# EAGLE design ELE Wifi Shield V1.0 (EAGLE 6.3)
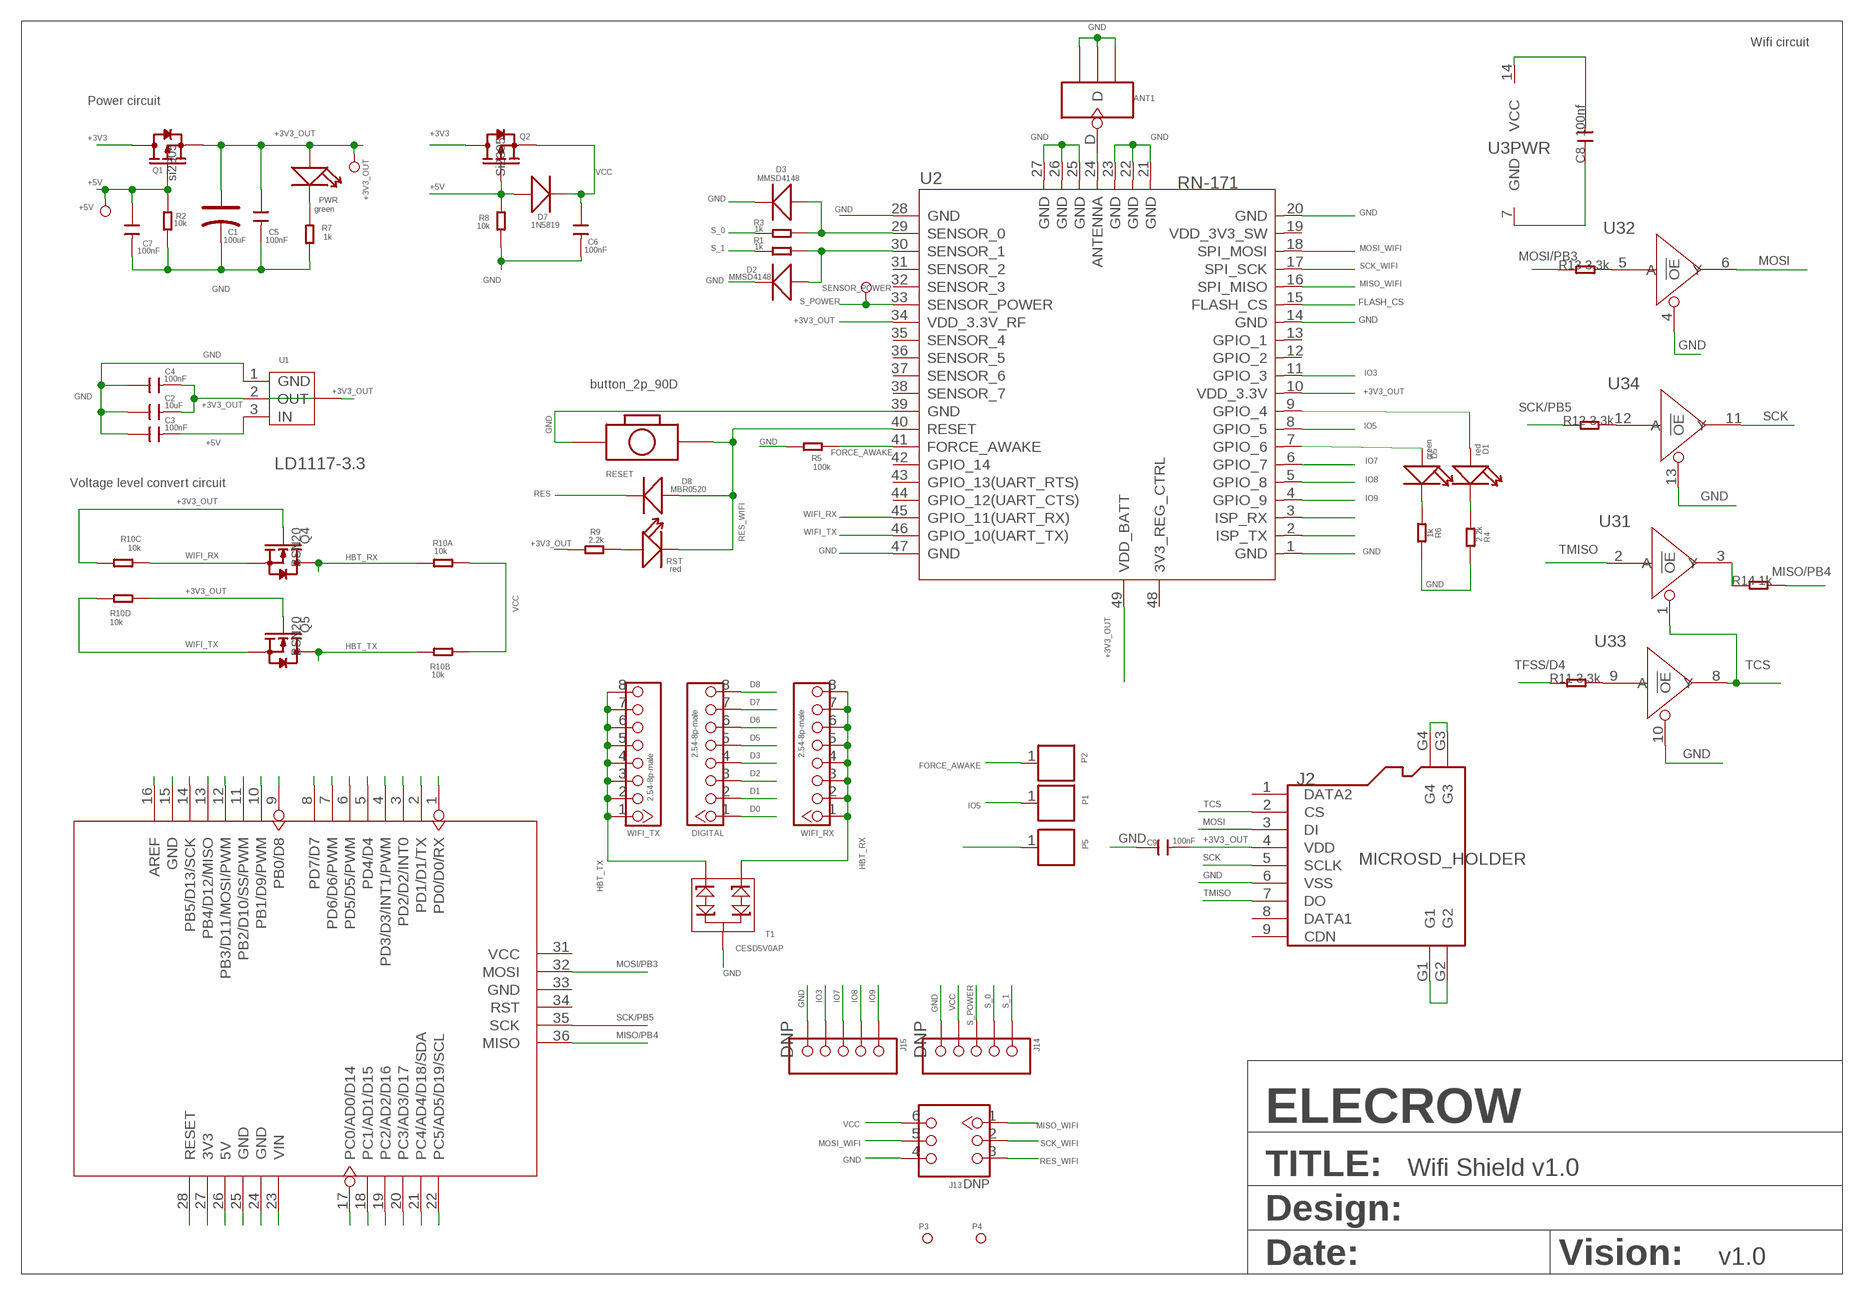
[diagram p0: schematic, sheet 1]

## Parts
+3V3_OUT  PAD-TEST-POINT-CIRCLE_SIZE_3030  [TP_3535]
+5V  PAD-TEST-POINT-CIRCLE_SIZE_3030  [TP_3535]
ANT1  ANTENNA-U-FL  [4P-U-FL]
C1  100uF  CAP-AVX-B  [AVX-B]
C2  10uF  C-0603  [C0603]
C3  100nF  C-0603  [C0603]
C4  100nF  C-0603  [C0603]
C5  100nF  C-0603  [C0603]
C6  100nF  C-0603  [C0603]
C7  100nF  C-0603  [C0603]
C8  100nf  C-0603  [C0603]
C9  100nF  C-0603  [C0603]
D1  red  LED'0603'  [LED-0603]
D2  MMSD4148  D-MBR0520LT1  [SOD123-2.7X1.6]
D3  MMSD4148  D-MBR0520LT1  [SOD123-2.7X1.6]
D5  green  LED'0603'  [LED-0603]
D7  1N5819  D-SMA  [D2010]
D8  MBR0520  D-MBR0520LT1  [SOD123-2.7X1.6]
DIGITAL  2.54-8p-male  HEADER-8P-2.54  [8P-2.54]
J2  MICROSD_HOLDER  HOLDER-MICROSD-9P  [9P-SMD-W/-RING]
J13  DNP  HEADER-2X3P-2.54  [2X3P-2.54]
J14  DNP  HEADER-5P-2.54  [5P-2.54]
J15  DNP  HEADER-5P-2.54  [5P-2.54]
P1  DNP  PAD'60/30'  [1P-65/35MIL]
P2  DNP  PAD'60/30'  [1P-65/35MIL]
P3  PAD-MARK  [ROUND-MARK-1.0]
P4  PAD-MARK  [ROUND-MARK-1.0]
P5  DNP  PAD'60/30'  [1P-65/35MIL]
PWR  green  LED'0603'  [LED-0603]
Q1  si2305  MOSFET-P'SI2323CDS/SI2305DS<BR>'  [SOT23]
Q2  Si2305  MOSFET-P'SI2323CDS/SI2305DS<BR>'  [SOT23]
Q4  BSN20  MOSFET-N'SOT23'  [SOT23]
Q5  BSN20  MOSFET-N'SOT23'  [SOT23]
R1  1k  R-0603  [R0603]
R2  10k  R-0603  [R0603]
R3  1k  R-0603  [R0603]
R4  2.2k  R-0603  [R0603]
R5  100k  R-0603  [R0603]
R6  1k  R-0603  [R0603]
R7  1k  R-0603  [R0603]
R8  10k  R-0603  [R0603]
R9  2.2k  R-0603  [R0603]
R10  10k  005-4R_1206  [R1206-8]
R11  3.3k  R-0603  [R0603]
R12  3.3k  R-0603  [R0603]
R13  3.3k  R-0603  [R0603]
R14  1k  R-0603  [R0603]
RESET  button_2p_90D  BOTTON-2P-90  [2P-7.62X3.56-90D]
RST  red  LED'0603'  [LED-0603]
SENSOR_POWER  PAD-TEST-POINT-CIRCLE_SIZE_3030  [TP_3535]
T1  CESD5V0AP  D-ESD-PESDXL2BT  [SOT23]
U1  LD1117-3.3  LD1117SOT89  [SOT89]
U2  RN-171  WIFI-RN-171  [49P-1.27-26.67X17.78]
U3  74VHC125PW  [TSSOP14]
U4  long female pin_8*2_6*2_2X3  ARDUINO  [ARDUINO]
WIFI_RX  2.54-8p-male  HEADER-8P-2.54  [8P-2.54]
WIFI_TX  2.54-8p-male  HEADER-8P-2.54  [8P-2.54]

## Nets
+3V3: Q1.3(D) Q2.3(D) U4.27(3V3)
+3V3_OUT: +3V3_OUT.T C1.+ C2.2 C4.2 C5.1 C9.2 J2.4(VDD) PWR.+ Q1.2(S) Q4.1(G) Q5.1(G) R9.2 R10.5 R10.6 U1.2(OUT) U1.4(TAB) U2.10(VDD_3.3V) U2.34(VDD_3.3V_RF) U2.49(VDD_BATT)
+5V: +5V.T C3.2 C7.1 D7.+ Q1.1(G) Q2.1(G) R2.1 R8.1 U1.3(IN) U4.26(5V)
A0: U4.17(PC0/AD0/D14)
A1: U4.18(PC1/AD1/D15)
A2: U4.19(PC2/AD2/D16)
A3: U4.20(PC3/AD3/D17)
A4: U4.21(PC4/AD4/D18/SDA)
A5: U4.22(PC5/AD5/D19/SCL)
AREF: U4.16(AREF)
D0: DIGITAL.1 U4.1(PD0/D0/RX)
D1: DIGITAL.2 U4.2(PD1/D1/TX)
D2: DIGITAL.3 U4.3(PD2/D2/INT0)
D3: DIGITAL.4 U4.4(PD3/D3/INT1/PWM)
D5: DIGITAL.5 U4.6(PD5/D5/PWM)
D6: DIGITAL.6 U4.7(PD6/D6/PWM)
D7: DIGITAL.7 U4.8(PD7/D7)
D8: DIGITAL.8 U4.9(PB0/D8)
D9: U4.10(PB1/D9/PWM)
D10: U4.11(PB2/D10/SS/PWM)
D11: U4.12(PB3/D11/MOSI/PWM)
D12: U4.13(PB4/D12/MISO)
D13: U4.14(PB5/D13/SCK)
FLASH_CS: P5.1 U2.15(FLASH_CS)
FORCE_AWAKE: P2.1 R5.1 U2.41(FORCE_AWAKE)
GND: ANT1.GND1 ANT1.GND2 ANT1.GND3 C1.- C2.1 C3.1 C4.1 C5.2 C6.2 C7.2 C8.1 C9.1 D2.1(-) D3.1(-) J2.6(VSS) J2.G1 J2.G2 J2.G3 J2.G4 J13.4 J14.5 J15.5 R2.2 R4.1 R5.2 R6.1 R7.1 R8.2 RESET.P$2 T1.3 U1.1(GND) U2.1(GND) U2.14(GND) U2.20(GND) U2.21(GND) U2.22(GND) U2.23(GND) U2.25(GND) U2.26(GND) U2.27(GND) U2.28(GND) U2.39(GND) U2.47(GND) U3.4(2:!OE) U3.7(PWR:GND) U3.10(3:!OE) U3.13(4:!OE) U4.15(GND) U4.24(GND) U4.25(GND)
HBT_RX: Q4.3(D) R10.1 T1.1 WIFI_RX.1 WIFI_RX.2 WIFI_RX.3 WIFI_RX.4 WIFI_RX.5 WIFI_RX.6 WIFI_RX.7 WIFI_RX.8
HBT_TX: Q5.3(D) R10.2 T1.2 WIFI_TX.1 WIFI_TX.2 WIFI_TX.3 WIFI_TX.4 WIFI_TX.5 WIFI_TX.6 WIFI_TX.7 WIFI_TX.8
IO3: J15.4 U2.11(GPIO_3)
IO5: P1.1 U2.8(GPIO_5)
IO7: J15.3 U2.6(GPIO_7)
IO8: J15.2 U2.5(GPIO_8)
IO9: J15.1 U2.4(GPIO_9)
MISO/PB4: R14.2 U4.36(MISO)
MISO_WIFI: J13.1 U2.16(SPI_MISO)
MOSI: J2.3(DI) U3.6(2:Y)
MOSI/PB3: R13.1 U4.32(MOSI)
MOSI_WIFI: J13.5 U2.18(SPI_MOSI)
N$1: R9.1 RST.+
N$2: D3.2(+) R3.1 U2.29(SENSOR_0)
N$3: D2.2(+) R1.1 U2.30(SENSOR_1)
N$6: R13.2 U3.5(2:A)
N$8: R12.2 U3.12(4:A)
N$10: U2.2(ISP_TX)
N$11: U2.3(ISP_RX)
N$12: R11.2 U3.9(3:A)
N$15: D5.+ U2.7(GPIO_6)
N$16: R14.1 U3.3(1:Y)
N$20: ANT1.D U2.24(ANTENNA)
N$22: D1.+ U2.9(GPIO_4)
N$23: D5.- R6.2
N$25: D1.- R4.2
N$26: PWR.- R7.2
RES: D8.1(-) U4.28(RESET)
RES_WIFI: D8.2(+) J13.3 RESET.P$1 RST.- U2.40(RESET)
S_0: J14.2 R3.2
S_1: J14.1 R1.2
S_POWER: J14.3 SENSOR_POWER.T U2.33(SENSOR_POWER)
SCK: J2.5(SCLK) U3.11(4:Y)
SCK/PB5: R12.1 U4.35(SCK)
SCK_WIFI: J13.2 U2.17(SPI_SCK)
TCS: J2.2(CS) U3.1(1:!OE) U3.8(3:Y)
TFSS/D4: R11.1 U4.5(PD4/D4)
TMISO: J2.7(DO) U3.2(1:A)
VCC: C6.1 C8.2 D7.- J13.6 J14.4 Q2.2(S) R10.7 R10.8 U3.14(PWR:VCC)
VIN: U4.23(VIN)
WIFI_RX: Q4.2(S) R10.3 U2.45(GPIO_11(UART_RX))
WIFI_TX: Q5.2(S) R10.4 U2.46(GPIO_10(UART_TX))
Unconnected: J2.1(DATA2) J2.8(DATA1) J2.9(CDN) U2.12(GPIO_2) U2.13(GPIO_1) U2.19(VDD_3V3_SW) U2.31(SENSOR_2) U2.32(SENSOR_3) U2.35(SENSOR_4) U2.36(SENSOR_5) U2.37(SENSOR_6) U2.38(SENSOR_7) U2.42(GPIO_14) U2.43(GPIO_13(UART_RTS)) U2.44(GPIO_12(UART_CTS)) U2.48(3V3_REG_CTRL) U4.31(VCC) U4.33(GND) U4.34(RST)

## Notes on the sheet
- Wifi circuit
- Power circuit
- Voltage level convert circuit
- ELECROW
- TITLE: | Wifi Shield v1.0
- Design:
- Date: | Vision: | v1.0

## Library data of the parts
+3V3_OUT +5V SENSOR_POWER = Discrete:PAD-TEST-POINT-CIRCLE
ANT1 = Connector:ANTENNA-U-FL
C1 = Discrete:CAP*: Electrolytic Capacitors,Tantalum Capacitors and Super Capacitors
C2-C9 = Discrete:C*: Ceramic Capacitors
D1 D5 PWR RST = Discrete:LED*
D2 D3 D7 D8 = Discrete:D*
DIGITAL WIFI_RX WIFI_TX = Connector:HEADER-8P
J2 = Connector:HOLDER-MICROSD-9P
J13 = Connector:HEADER-2X3P
J14 J15 = Connector:HEADER-5P
P1 P2 P5 = Discrete:PAD
P3 P4 = Discrete:PAD-MARK; PARTNO: DNP
Q1 Q2 = Discrete:MOSFET-P
Q4 Q5 = Discrete:MOSFET-N: IRLL014: http://www.vishay.com/docs/91319/sihll014.pdf
R1-R9 R11-R14 = Discrete:R*
R10 = Discrete:005-4R*: Resistor Array
RESET = Discrete:BOTTON-2P
T1 = Discrete:D-ESD-PESDXL2BT
U1 = IC:LD1117: Low Drop Fixed And Adjustable Positive Voltage Regulators http://www.datasheetcatalog.org/datasheet/SGSThomsonMicroelectronics/mXuqtqv.pdf
U2 = Module:WIFI-RN-171: WIFLY GSX 802.11 b/g wireless LAN Module
U3 = template:74V*125: Quad Buffer/Line Driver;3-state
U4 = moudle:ARDUINO

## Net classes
0 default: width 0.003 mm, drill 0.254 mm, clearance 0.152 mm

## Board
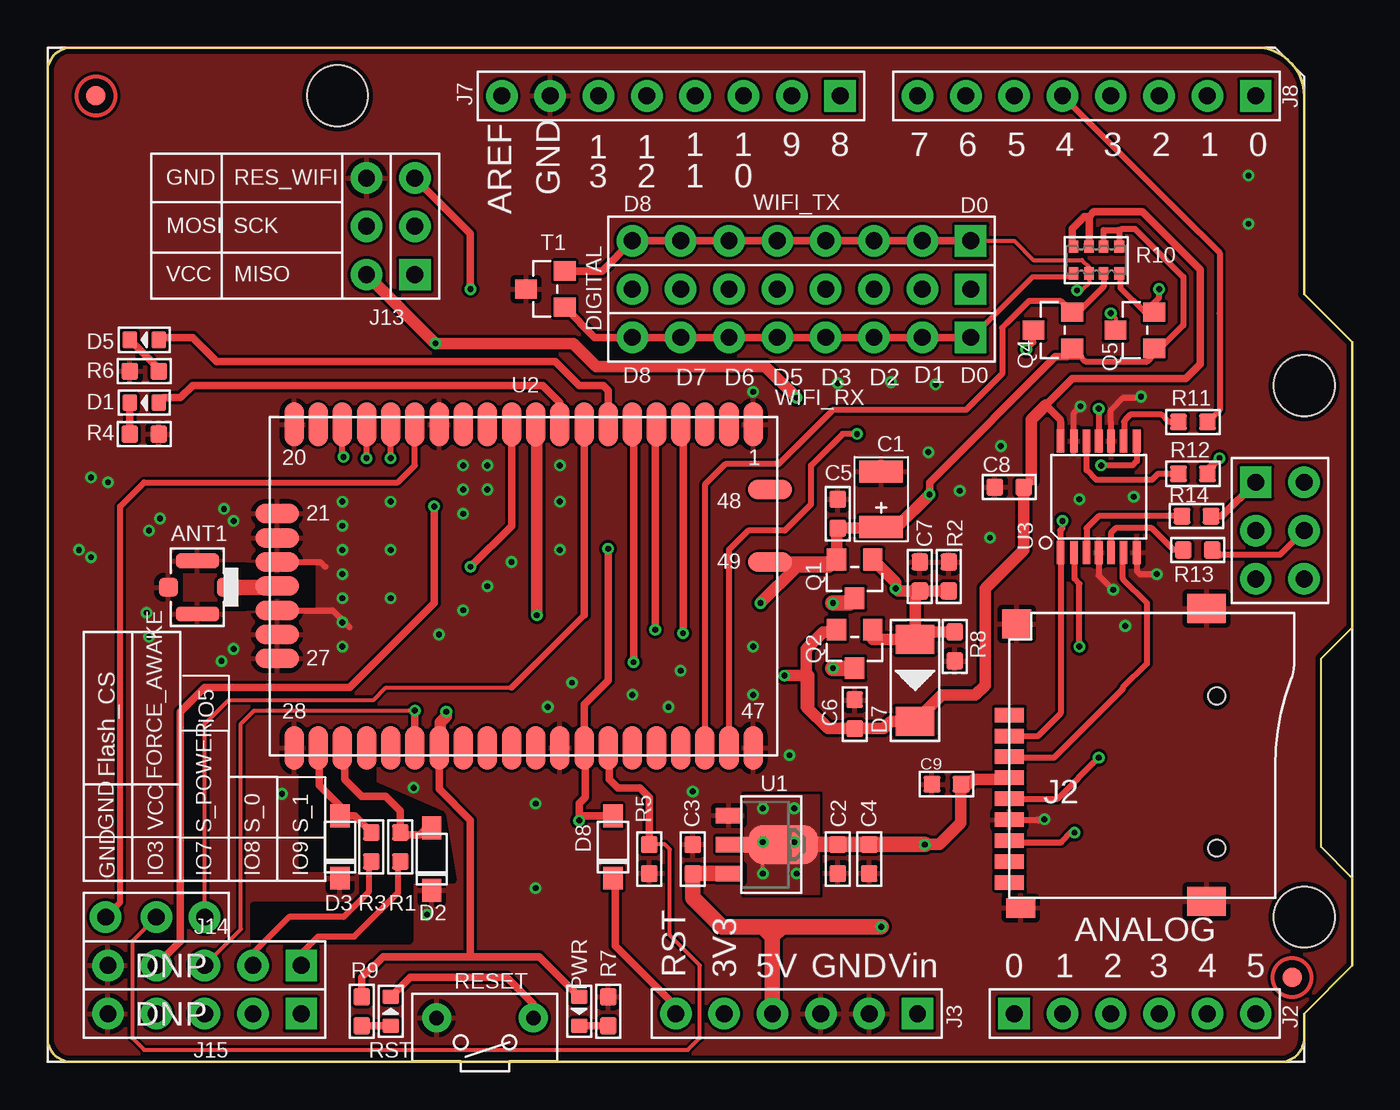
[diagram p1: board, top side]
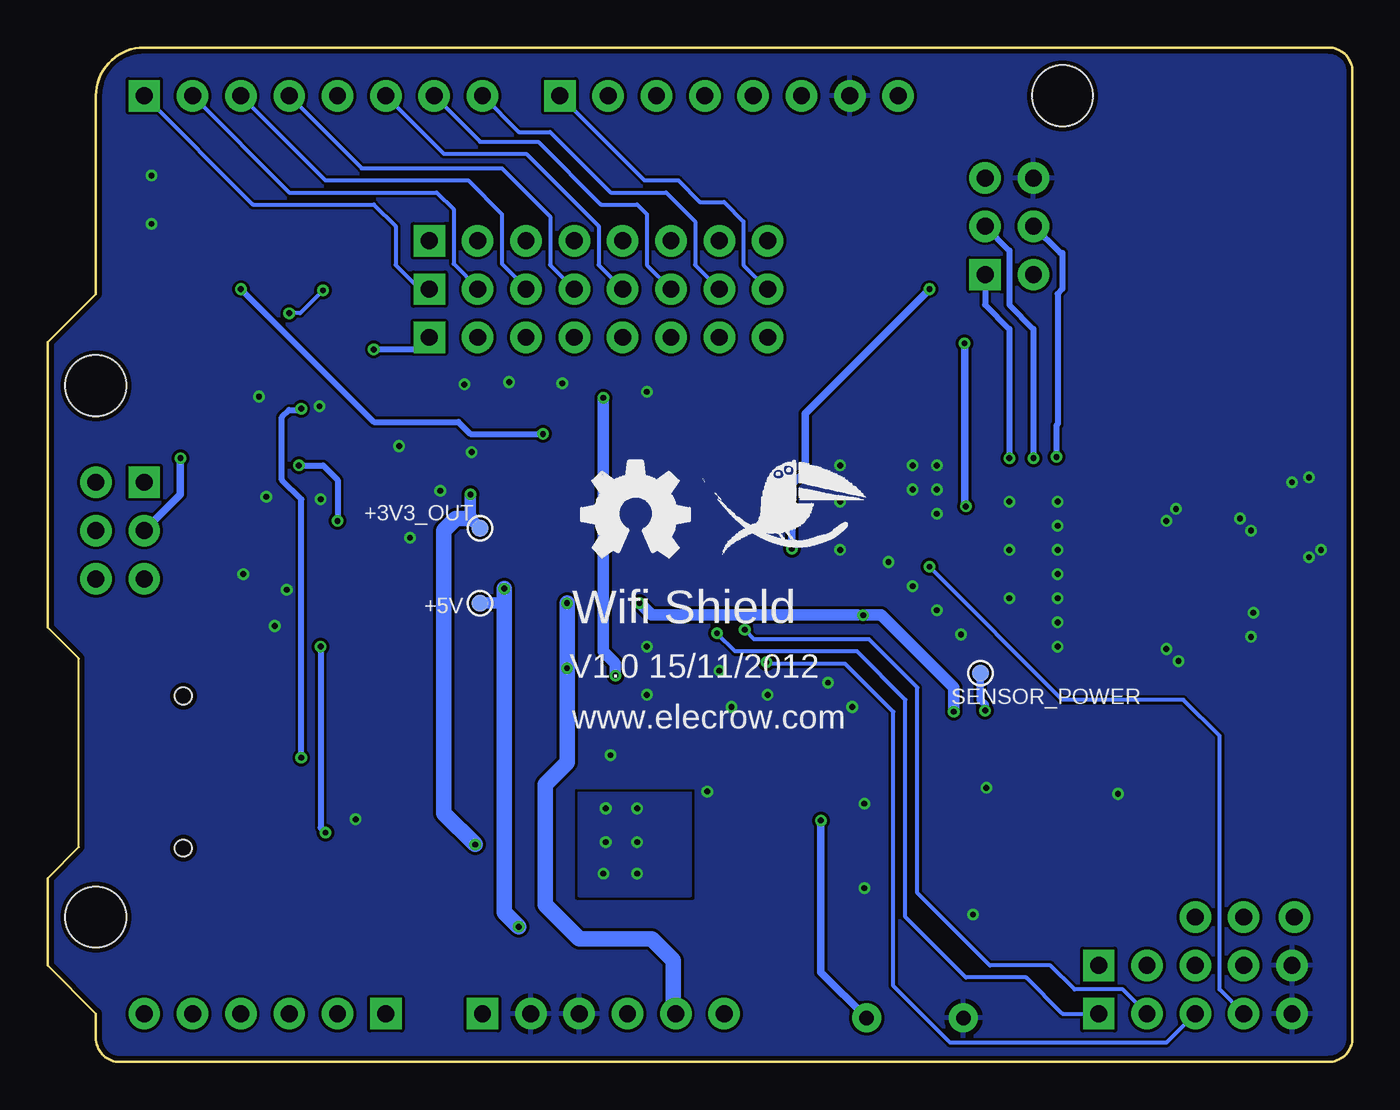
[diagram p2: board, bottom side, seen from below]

Size 68.58 x 53.34 mm. Coordinates in mm from the lower left corner, seen from the top.
Outline: 1.27,53.34 63.5,53.34 arc-90 66.04,50.8 66.04,40.39 68.58,37.85 68.58,22.86 66.93,21.21 66.93,11.3 68.58,9.65 68.58,5.08 66.04,2.54 66.04,1.27 arc-90 64.77,0 1.27,0 arc-90 0,1.27 0,52.07 arc-90 1.27,53.34
Copper layers (1*16): Top 0.035mm / dielectric 1.5mm / Bottom 0.035mm
Design rules "default": minimum track width 6mil, minimum drill 12mil, track to track 6mil, track to pad 6mil, pad to pad 6mil, via to via 6mil, smd to smd 0mil, copper to edge 10mil, drill to drill 10mil, minimum pad ring 10mil, minimum via ring 6mil, stop-mask expansion 2mil, vias tented up to drill 32mil, thermal gap 10mil
tRestrict: 16 lines

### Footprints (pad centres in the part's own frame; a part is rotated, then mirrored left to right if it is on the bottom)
TP_3535 = smd 0.889 x 0.889: T 0,0
4P-U-FL = smd 1.016 x 1.016: D -1.524,0; GND3 1.524,0 | smd 2.286 x 0.762: GND1 0,1.397; GND2 0,-1.397
AVX-B = smd 1.143 x 2.286: + -1.46,0; - 1.46,0
C0603 = smd 0.889 x 0.889: 1 -0.762,0; 2 0.762,0
LED-0603 = smd 0.762 x 0.889: + -0.762,0; - 0.762,0
SOD123-2.7X1.6 = smd 1.2 x 1.02: 1 -1.635,0; 2 1.635,0
D2010 = smd 1.524 x 2.032: + -2.159,0; - 2.159,0
8P-2.54 = drill 0.889 pad 1.651 square: 1 0,8.89 | drill 0.889 pad 1.651: 2 0,6.35; 3 0,3.81; 4 0,1.27; 5 0,-1.27; 6 0,-3.81; 7 0,-6.35; 8 0,-8.89
9P-SMD-W/-RING = smd 1.524 x 0.762: 1 0,4.4; 2 0,3.3; 3 0,2.2; 4 0,1.1; 5 0,0; 6 0,-1.1; 7 0,-2.2; 8 0,-3.3; 9 0,-4.4 | smd 1.524 x 1.016: G1 0.6,-5.746 | smd 2.032 x 1.524: G2 10.373,-5.4; G3 10.373,10 | smd 1.524 x 1.524: G4 0.392,9.181 | hole 0.889: 10.9,-2.6; 10.9,5.4
2X3P-2.54 = drill 0.889 pad 1.651 square: 1 -1.27,2.54 | drill 0.889 pad 1.651: 2 -1.27,0; 3 -1.27,-2.54; 4 1.27,-2.54; 5 1.27,0; 6 1.27,2.54
5P-2.54 = drill 0.889 pad 1.651 square: 1 0,5.08 | drill 0.889 pad 1.651: 2 0,2.54; 3 0,0; 4 0,-2.54; 5 0,-5.08
1P-65/35MIL = drill 0.889 pad 1.651: 1 0,0
ROUND-MARK-1.0 = smd 1.016 x 1.016: P$1 0,0
SOT23 = smd 1.016 x 1.143: 1 -0.95,-1.016; 2 0.95,-1.016; 3 0,1.016
R0603 = smd 0.889 x 0.889: 1 -0.762,0; 2 0.762,0
R1206-8 = smd 0.508 x 0.635: 1 -1.206,-0.699; 2 -0.381,-0.699; 3 0.381,-0.699; 4 1.206,-0.699; 5 1.206,0.699; 6 0.381,0.699; 7 -0.381,0.699; 8 -1.206,0.699
2P-7.62X3.56-90D = drill 0.762 pad 1.524: P$1 0,2.54; P$2 0,-2.54
SOT89 = smd 0.8 x 1.4: 1 -1.524,-1.905; 3 1.524,-1.905 | smd 0.8 x 1.9: 2 0,-1.651 | smd 2.032 x 3.65: 4 0,0.94
49P-1.27-26.67X17.78 = smd 1.016 x 2.286: 1 12.065,8.509; 2 10.795,8.509; 3 9.525,8.509; 4 8.255,8.509; 5 6.985,8.509; 6 5.715,8.509; 7 4.445,8.509; 8 3.175,8.509; 9 1.905,8.509; 10 0.635,8.509; 11 -0.635,8.509; 12 -1.905,8.509; 13 -3.175,8.509; 14 -4.445,8.509; 15 -5.715,8.509; 16 -6.985,8.509; 17 -8.255,8.509; 18 -9.525,8.509; 19 -10.795,8.509; 20 -12.065,8.509; 28 -12.065,-8.509; 29 -10.795,-8.509; 30 -9.525,-8.509; 31 -8.255,-8.509; 32 -6.985,-8.509; 33 -5.715,-8.509; 34 -4.445,-8.509; 35 -3.175,-8.509; 36 -1.905,-8.509; 37 -0.635,-8.509; 38 0.635,-8.509; 39 1.905,-8.509; 40 3.175,-8.509; 41 4.445,-8.509; 42 5.715,-8.509; 43 6.985,-8.509; 44 8.255,-8.509; 45 9.525,-8.509; 46 10.795,-8.509; 47 12.065,-8.509 | smd 2.286 x 1.016: 21 -12.954,3.81; 22 -12.954,2.54; 23 -12.954,1.27; 24 -12.954,0; 25 -12.954,-1.27; 26 -12.954,-2.54; 27 -12.954,-3.81; 48 12.954,5.08; 49 12.954,1.27
TSSOP14 = smd 0.4 x 1.2: 1 -2,-2.925; 2 -1.3,-2.925; 3 -0.65,-2.925; 4 0,-2.925; 5 0.65,-2.925; 6 1.3,-2.925; 7 2,-2.925; 8 2,2.925; 9 1.3,2.925; 10 0.65,2.925; 11 0,2.925; 12 -0.65,2.925; 13 -1.3,2.925; 14 -2,2.925
ARDUINO = drill 0.889 pad 1.651 square: 1 63.5,50.8; 9 41.656,50.8; 17 50.8,2.54; 23 45.72,2.54; 36 63.5,30.48 | drill 0.889 pad 1.651: 2 60.96,50.8; 3 58.42,50.8; 4 55.88,50.8; 5 53.34,50.8; 6 50.8,50.8; 7 48.26,50.8; 8 45.72,50.8; 10 39.116,50.8; 11 36.576,50.8; 12 34.036,50.8; 13 31.496,50.8; 14 28.956,50.8; 15 26.416,50.8; 16 23.876,50.8; 18 53.34,2.54; 19 55.88,2.54; 20 58.42,2.54; 21 60.96,2.54; 22 63.5,2.54; 24 43.18,2.54; 25 40.64,2.54; 26 38.1,2.54; 27 35.56,2.54; 28 33.02,2.54; 31 66.04,30.48; 32 66.04,27.94; 33 66.04,25.4; 34 63.5,25.4; 35 63.5,27.94 | hole 3.2: 15.24,50.8; 66.04,35.56; 66.04,7.62

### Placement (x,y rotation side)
+3V3_OUT  45.85,28.07 180 bottom
+5V  45.85,24.13 0 bottom
ANT1  7.87,24.96 180 top
C1  43.81,29.59 90 top
C2  41.53,10.67 90 top
C3  33.91,10.67 270 top
C4  43.18,10.67 90 top
C5  41.53,28.83 90 top
C6  42.42,18.29 90 top
C7  45.85,25.53 90 top
C8  50.55,30.23 0 top
C9  47.24,14.61 0 top
D1  5.08,34.67 180 top
D2  20.19,10.67 90 top
D3  15.37,11.3 90 top
D5  5.08,37.97 180 top
D7  45.59,20.07 270 top
D8  29.72,11.3 90 top
DIGITAL  39.62,40.64 270 top
J2  50.55,13.84 0 top
J13  18.03,43.94 180 top
J14  8.26,5.08 270 top
J15  8.26,2.54 270 top
P1  8.26,7.62 0 top
P2  5.71,7.62 0 top
P3  2.54,50.8 0 top
P4  65.41,4.45 0 top
P5  3.05,7.62 0 top
PWR  27.94,2.67 270 top
Q1  42.42,25.4 180 top
Q2  42.42,21.72 180 top
Q4  52.83,38.48 90 top
Q5  57.15,38.48 90 top
R1  18.54,11.3 270 top
R2  47.37,25.53 90 top
R3  17.02,11.3 270 top
R4  5.08,33.02 180 top
R5  31.62,10.67 270 top
R6  5.08,36.32 0 top
R7  29.46,2.67 270 top
R8  47.68,21.84 270 top
R9  16.51,2.67 90 top
R10  55.12,42.16 0 top
R11  60.2,33.66 180 top
R12  60.2,30.92 180 top
R13  60.45,26.92 180 top
R14  60.39,28.7 0 top
RESET  22.99,2.31 270 top
RST  18.03,2.67 90 top
SENSOR_POWER  19.56,20.45 0 bottom
T1  26.16,40.64 90 top
U1  37.72,11.43 270 top
U2  25.02,25.02 0 top
U3  55.24,29.72 0 top
U4  0,0 0 top
U$1  [OSHW_FILLX200_NOTEXT]  40.51,26.54 0 bottom
U$3  [ELECROW4]  34.29,25.27 0 bottom
WIFI_RX  39.62,38.1 270 top
WIFI_TX  39.62,43.18 270 top

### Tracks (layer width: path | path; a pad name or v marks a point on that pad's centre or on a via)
+3V3  (via drill 0.3)
  Top 0.813: v41.27,24.13 42.16,24.13 Q1.3 | Q2.3 v41.27,20.7
  Bottom 0.813: U4.27 35.69,2.67 35.69,5.33 36.83,6.48 40.64,6.48 42.42,8.26 42.42,14.61 41.27,15.75 v41.27,20.7 v41.27,24.13
+3V3_OUT  (via drill 0.3)
  Top 0.203: v37.59,9.91 37.59,11.43 | U1.2 37.59,11.43 | 37.59,11.43 v37.59,11.56 | v39.24,11.56 38.73,11.56 38.73,11.43
  Top 0.305: R10.6 55.5,43.75 56.26,43.75 56.33,43.69 | 56.33,43.69 R10.5 | 56.33,43.69 56.45,43.81 57.15,43.81 59.69,41.27 59.69,38.73 58.49,37.53 Q5.1 58.17,37.21 57.78,36.83 54.55,36.83 54.26,37.12 Q4.1
  Top 0.406: 54.26,37.12 53.63,37.12 53.59,37.08 52.96,37.08 46.35,30.48 v46.35,29.84 | U2.49 38.23,26.04 38.73,26.04 | R9.2 16.51,4.45 17.14,5.08 17.21,5.08 17.65,5.52 22.23,5.52 | 22.23,5.52 25.84,5.52 PWR.+ | U2.34 20.57,14.35 22.23,12.7 22.23,5.52
  Top 0.457: U2.34 20.64,16.57
  Top 0.61: J2.4 50.46,14.86 48.64,14.86 48.39,14.61 C9.2 48.01,12.57 46.86,11.43 v46.1,11.43 | Q1.2 41.21,26.16 41.09,26.29 U2.49 | Q1.2 41.47,28.01 C5.1 43.75,28.07 C1.+ 44.64,28.13 v46.35,29.84 | Q1.2 41.09,26.04 39.37,26.04 v37.47,24.13 | 20.64,16.57 20.64,17.84 20.95,18.16 v20.95,18.41 | U2.10 25.72,33.47 v25.72,23.5
  Top 0.813: U1.4 38.73,11.43 C2.2 C4.2 v46.1,11.43
  Bottom 0.457: 26.04,23.5 v25.72,23.5
  Bottom 0.61: v46.35,29.84 46.35,28.57 +3V3_OUT.T | v37.47,24.13 36.83,23.5 26.04,23.5 | v25.72,23.5 24.77,23.5 20.95,19.68 v20.95,18.41
  Bottom 0.813: v46.1,11.43 47.75,13.08 47.75,27.94 47.12,28.57 46.35,28.57
  other vias: 37.59,13.34 39.24,13.34 39.37,9.91
  pour Top (isolate 0.254, no thermals): 40.51,13.97 36.7,13.97 36.7,8.89 40.51,8.89
  pour Bottom (isolate 0.254, no thermals): 34.86,13.53 34.86,13.97 40.64,13.97 40.64,8.89 34.92,8.89
+5V  (via drill 0.3)
  Top 0.61: Q1.1 44.58,25.21 v44.58,24.89 44.7,24.77 C7.1 | C7.1 45.59,24.51 D7.+ | D7.+ 45.97,22.61 R8.1 | D7.+ 43.37,22.23 Q2.1 | R2.1 C7.1
  Top 0.813: U4.26 38.1,6.6 | 38.1,6.6 37.59,7.11 | 37.59,7.11 35.43,7.11 33.91,8.64 C3.2 U1.3 | 37.59,7.11 38.61,7.11 | 38.1,6.6 38.61,7.11 | 38.61,7.11 v43.81,7.11
  Bottom 0.61: +5V.T 44.83,24.13 44.58,24.38
  Bottom 0.813: v44.58,24.89 44.58,24.38 44.58,7.87 v43.81,7.11
D0
  Bottom 0.203: U4.1 57.78,45.09 51.44,45.09 50.29,43.94 50.29,41.91 49.02,40.64 DIGITAL.1
D1
  Bottom 0.203: U4.2 55.88,45.72 48.13,45.72 47.24,44.83 47.24,41.97 45.97,40.7 DIGITAL.2
D2
  Bottom 0.203: U4.3 53.98,46.35 46.48,46.35 44.7,44.58 44.7,41.97 43.43,40.7 DIGITAL.3
D3
  Bottom 0.203: U4.4 52.07,46.99 44.7,46.99 42.16,44.45 42.16,41.91 DIGITAL.4
D5
  Bottom 0.203: U4.6 47.75,47.75 43.43,47.75 39.62,43.94 39.62,41.91 DIGITAL.5
D6
  Bottom 0.203: U4.7 45.85,48.39 42.8,48.39 39.5,45.09 37.59,45.09 37.08,44.58 37.08,41.91 DIGITAL.6
D7
  Bottom 0.203: U4.8 43.81,48.9 42.16,48.9 38.99,45.72 36.07,45.72 34.54,44.2 34.54,41.91 DIGITAL.7
D8
  Bottom 0.203: U4.9 37.21,46.35 35.43,46.35 34.29,45.21 33.02,45.21 32,44.2 32,41.91 DIGITAL.8
FLASH_CS
  Top 0.305: P5.1 3.81,8.38 3.81,29.21 5.08,30.48 18.41,30.48 19.3,31.37 U2.15
FORCE_AWAKE
  Top 0.203: P2.1 4.45,6.35 4.45,1.27 5.08,0.64 33.66,0.64 34.29,1.27 34.29,5.08 32.7,6.67 32.7,11.18 32.45,11.43 R5.1
  Top 0.406: U2.41 29.53,16.45 29.53,14.86 29.97,14.41 31.11,14.41 31.62,13.91 R5.1
GND  (via drill 0.3)
  Top 0.305: U3.4 55.24,25.59 v56.01,24.83 | J2.6 52.03,12.74 52.07,12.7 | U2.23 14.35,26.29 14.61,26.04 | U2.25 14.99,23.75 15.88,22.86 | U3.10 55.9,33.64 55.88,33.66 55.88,34.29 56.52,34.92 57.15,34.92 | U3.13 53.95,34.13 v54.29,34.48 | U3.7 57.24,25.81 57.4,25.65 v58.29,25.65
  other vias: 2.29,26.54 5.91,28.57 9.27,29.08 9.78,28.45 3.17,30.48 1.65,26.92 15.49,29.46 2.29,30.73 5.33,27.94 5.21,23.62 5.33,22.35 9.14,21.08 9.78,21.72 15.49,28.19 15.49,26.92 15.49,25.65 15.49,24.38 15.49,23.11 15.49,21.84 21.84,31.37 23.11,31.37 23.11,30.1 21.84,30.1 21.84,28.83 24.38,26.29 23.11,25.02 21.84,23.75 20.57,22.48 26.92,31.37 26.92,29.46 26.92,26.92 33.27,20.57 30.73,19.3 32.64,18.67 27.56,19.94 26.29,18.67 37.08,21.84 37.08,19.3 25.65,13.59 25.65,9.14 18.03,29.46 18.03,26.92 18.03,24.38 63.12,46.61 63.12,44.07 52.39,12.76 57.09,29.72 54.23,29.59 56.64,22.92 57.47,34.99 50.1,32.38 46.29,32.07 46.67,35.62 44.32,35.75 41.53,35.69 47.94,30.04 49.53,27.56 33.91,14.22 38.99,16.13 37.08,35.24 12.32,14.1 19.94,7.75 19.24,14.41
  pour Bottom: -10.16,34.67 -5.84,34.67 -5.84,30.35 -10.16,30.35
  pour Bottom (rank 6): 0,0 68.58,0 68.58,53.34 0,53.34
  pour Top (rank 6): 0,53.34 0,0.64 arc90 0.64,0 66.78,0 arc90 68.58,1.8 68.58,50.5 arc90 65.74,53.34
HBT_RX  (via drill 0.3)
  Top 0.254: WIFI_RX.1 48.58,38.1 51.75,41.27 53.72,41.27 R10.1
  Top 0.305: 51.44,38.1 Q4.3 51.82,37.85 v51.44,37.47
  Top 0.406: T1.1 28.77,38.1 WIFI_RX.8 WIFI_RX.7 WIFI_RX.6 WIFI_RX.5 WIFI_RX.4 WIFI_RX.3 WIFI_RX.2 WIFI_RX.1
  Bottom 0.305: WIFI_RX.1 49.15,37.47 v51.44,37.47
HBT_TX  (via drill 0.3)
  Top 0.203: WIFI_TX.1 50.8,43.18 51.82,42.16 54.36,42.16 54.74,41.78 R10.2 54.61,41.34 54.61,41.27 54.74,41.15 54.74,40.96 54.36,40.58 v54.1,40.58 | v55.88,39.37 56.13,39.12 Q5.3
  Top 0.406: T1.2 29.14,41.59 WIFI_TX.8 WIFI_TX.7 WIFI_TX.6 WIFI_TX.5 WIFI_TX.4 WIFI_TX.3 WIFI_TX.2 WIFI_TX.1
  Bottom 0.203: v54.1,40.58 55.31,39.37 v55.88,39.37
IO3  (via drill 0.3)
  Top 0.406: v22.23,26.04 24.38,28.19 U2.11
  Bottom 0.203: J15.4 6.99,3.81 6.99,17.14 8.89,19.05 15.24,19.05 v22.23,26.04
IO5
  Top 0.203: P1.1 8.26,17.78 9.53,19.05 17.14,19.05 17.78,19.68 24.38,19.68
  Top 0.305: 28.19,23.5 24.38,19.68
  Top 0.406: 28.32,33.4 U2.8 28.19,23.5
IO7  (via drill 0.3)
  Top 0.406: U2.6 30.8,33.47 v30.8,21.02
  Bottom 0.203: J15.3 9.78,1.02 21.14,1.02 24.13,4 24.13,18.41 26.67,20.95 30.73,20.95 v30.8,21.02
IO8  (via drill 0.3)
  Top 0.406: U2.5 31.94,33.47 v31.94,22.73
  Bottom 0.203: J15.2 12.06,3.81 14.61,3.81 15.88,5.08 19.05,5.08 22.86,8.89 22.86,19.68 25.4,22.23 31.43,22.23 v31.94,22.73
IO9  (via drill 0.3)
  Top 0.406: U2.4 33.4,33.4 v33.4,22.54
  Bottom 0.203: J15.1 15.24,2.54 17.14,4.45 20.32,4.45 23.5,7.62 23.5,19.05 26.04,21.59 32.45,21.59 v33.4,22.54
MISO/PB4
  Top 0.406: U4.36 61.72,28.7 R14.2
MISO_WIFI  (via drill 0.3)
  Top 0.305: v18.03,31.75 U2.16
  Bottom 0.305: J13.1 19.3,39.81 18.03,38.54 v18.03,31.75
MOSI
  Top 0.305: 50.59,16 52.9,16 56.52,19.62 56.52,19.68 57.78,20.95 57.78,24.13 56.52,25.4 56.52,26.76 U3.6
  Top 0.406: J2.3 50.59,16
MOSI/PB3
  Top 0.305: U4.32 64.77,26.67 61.59,26.67
  Top 0.406: 61.59,26.67 61.34,26.92 R13.1
MOSI_WIFI  (via drill 0.3)
  Top 0.305: v15.56,31.81 15.49,31.88 U2.18
  Bottom 0.305: J13.5 15.37,42.55 15.24,42.55 15.24,40.64 15.49,40.39 U2.18 15.56,33.47 v15.56,31.81
N$1
  Top 0.406: R9.1 RST.+
N$2
  Top 0.406: U2.29 14.29,16.45 14.29,14.54 15.37,13.46 D3.2 16.14,12.94 R3.1
N$3
  Top 0.254: R1.1 18.67,11.94 | 19.8,12.3 D2.2
  Top 0.406: U2.30 15.62,16.38 15.62,14.86 16.51,13.97 17.78,13.97 18.54,13.21 R1.1 | 18.67,11.94 19.56,11.94 19.92,12.3 D2.2
N$4
  pour Bottom: 34.8,14.1 40.64,14.1 40.64,8.76 34.8,8.76
N$6
  Top 0.254: 55.88,26.81 U3.5
  Top 0.305: R13.2 59.18,26.92 58.04,28.07 56.13,28.07 55.88,27.81 55.88,26.81
N$8
  Top 0.254: 54.61,32.63 U3.12
  Top 0.305: R12.2 58.36,30.92 58.04,30.61 55.12,30.61 54.61,31.11 54.61,32.63
N$12
  Top 0.254: 56.64,33.78 56.64,33.72 56.58,33.66 | 56.58,32.68 U3.9
  Top 0.305: R11.2 58.93,33.66 58.55,34.04 56.9,34.04 56.64,33.78 | 56.58,33.66 56.58,32.68
N$15
  Top 0.406: D5.+ 5.97,38.1 7.62,38.1 8.89,36.83 26.67,36.83 27.94,35.56 29.21,35.56 29.46,35.31 U2.7
N$16
  Top 0.254: 54.61,26.81 U3.3
  Top 0.305: R14.1 55.24,28.7 54.61,28.07 54.61,26.81
N$20
  Top 0.813: U2.24 12,24.96 ANT1.D
N$22
  Top 0.406: 27.05,33.4 U2.9 26.92,34.67 26.04,35.56 7.62,35.56 6.99,34.92 6.1,34.92 D1.+
N$23
  Top 0.406: D5.- 5.84,36.45 R6.2
N$25
  Top 0.406: D1.- R4.2
N$26
  Top 0.406: R7.2 PWR.-
RES
  Top 0.406: D8.1 29.84,9.54 29.84,6.1 33.02,2.92 U4.28
RES_WIFI  (via drill 0.3)
  Top 0.406: RESET.P$1 25.53,3.05 24.13,4.45 19.05,4.45 RST.- | D8.2 28.18,12.94 v27.94,12.7 27.94,13.59 28.26,13.91 28.26,16.45 U2.40 28.19,18.8 29.46,20.07 v29.46,26.99 | J13.3 22.23,43.56 v22.23,40.64
  Bottom 0.406: v27.94,12.7 27.94,4.72 RESET.P$1 | v22.23,40.64 28.77,34.1 28.77,31.05 29.46,30.35 v29.46,26.99
S_0
  Top 0.305: R3.2 16.89,10.41 16.89,8.95 15.56,7.62 12.7,7.62 10.79,5.71 J14.2
S_1
  Top 0.305: R1.2 18.41,10.41 18.41,8.89 16.13,6.6 14.22,6.6 13.34,5.71 J14.1
S_POWER  (via drill 0.3)
  Top 0.203: J14.3 10.16,6.99 10.16,17.78 10.86,18.48 v19.3,18.48
  Top 0.406: 19.37,16.57 U2.33 v19.3,18.48
  Bottom 0.406: SENSOR_POWER.T 19.56,19.05 19.3,18.8 v19.3,18.48
SCK  (via drill 0.3)
  Top 0.305: J2.5 53.09,13.84 v55.24,16 | v55.24,34.35 U3.11
  Bottom 0.305: v55.24,16 55.24,29.59 56.26,30.61 56.26,33.91 55.88,34.29 55.31,34.29 v55.24,34.35
SCK/PB5  (via drill 0.3)
  Top 0.406: v61.59,31.75 60.96,31.11 R12.1
  Bottom 0.406: U4.35 61.59,29.84 v61.59,31.75
SCK_WIFI  (via drill 0.3)
  Top 0.305: v16.76,31.75 U2.17
  Bottom 0.305: J13.2 18.03,42.67 18.03,39.81 16.76,38.54 v16.76,31.75
TCS  (via drill 0.3)
  Top 0.254: 53.21,26.82 U3.1
  Top 0.305: J2.2 52.07,17.14 52.7,17.78 53.24,18.32 U3.1 | U3.8 57.24,31.59 57.02,31.37 v55.37,31.37 | v53.34,28.45 53.34,28.07 53.21,27.94 53.21,26.82
  Top 0.406: J2.2
  Bottom 0.305: v55.37,31.37 54.1,31.37 53.34,30.61 v53.34,28.45
TFSS/D4
  Top 0.305: U4.5 59.56,44.58 61.59,42.55 61.59,39.37 61.59,34.29 R11.1
TMISO  (via drill 0.3)
  Top 0.254: 53.98,26.76 U3.2 | v53.98,12.06 53.78,12.06
  Top 0.305: 50.63,11.56 53.28,11.56 53.78,12.06 | v54.23,21.84 54.23,25.15 53.98,25.4 53.98,26.76
  Top 0.406: J2.7 50.63,11.56
  Bottom 0.305: v54.23,21.84 54.23,12.32 v53.98,12.06
VCC  (via drill 0.3)
  Top 0.254: 51.69,30.61 C8.2 | 53.24,33.62 53.21,33.66 53.21,33.78
  Top 0.305: R10.7 54.61,42.99
  Top 0.406: 53.98,42.93 R10.8 53.85,42.93 53.85,43.81 54.48,44.45 54.74,44.45 | R10.7 54.74,44.45 | 54.74,44.45 54.99,44.7 57.53,44.7 60.58,41.66 60.58,36.7 59.82,35.94 53.85,35.94 52.45,34.54 53.21,33.78 | J14.4 6.99,6.35 6.99,17.14 6.99,18.41 8.26,19.68 15.88,19.68 17.14,20.95 20.32,24.13 v20.32,29.21 | U3.14 53.24,33.62
  Top 0.61: 39.88,18.67 41.02,17.53 C6.1 43.94,17.53 44.32,17.91 D7.- 46.99,19.3 48.77,19.3 49.28,19.81 49.28,24.89 51.31,26.92 C8.2 | 39.88,18.67 39.88,21.72 40.77,22.61 41.34,22.61 Q2.2 | 39.88,18.67 40.01,18.8 40.01,20.32 v38.73,20.32 | v39.37,34.92 37.72,36.58 28.83,36.58 27.62,37.78 v20.38,37.78 J13.6 | 52.45,34.54 51.69,33.78 51.69,30.61
  Bottom 0.406: v20.32,29.21 20.38,29.27 v20.38,37.78
  Bottom 0.61: v39.37,34.92 39.37,21.59 38.73,20.95 v38.73,20.32
WIFI_RX
  Top 0.254: 50.42,38.86 50.16,38.61
  Top 0.305: R10.3 55.5,40.77 54.16,39.43 Q4.2 53.27,40.01 51.56,40.01 50.42,38.86 | U2.45 34.54,30.35 35.62,31.43 38.42,31.43 41.27,34.29 48.26,34.29 50.16,36.2 50.16,38.61
WIFI_TX  (via drill 0.3)
  Top 0.305: R10.4 56.39,41.4 56.39,40.7 57.66,39.43 | 57.66,39.43 Q5.2 | 57.66,39.43 58.42,40.19 v58.42,40.64 | v42.55,33.02 41.78,33.02 40.13,31.37 40.13,29.34 38.73,27.94 36.83,27.94 35.81,26.92 U2.46
  Bottom 0.305: v58.42,40.64 51.44,33.66 46.99,33.66 46.35,33.02 v42.55,33.02

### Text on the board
tPlace: J7 | J8 | GND | RES_WIFI | D8 | D0 | MOSI | SCK | VCC | MISO | D8 | D7 | D6 | D5 | D3 | D2 | D1 | D0 | IO5 | Flash_CS | FORCE_AWAKE | GND | VCC | S_POWER | S_0 | S_1 | GND | IO3 | IO7 | IO8 | IO9 | J3 | J2
bPlace: Wifi Shield | V1.0 15/11/2012 | www.elecrow.com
